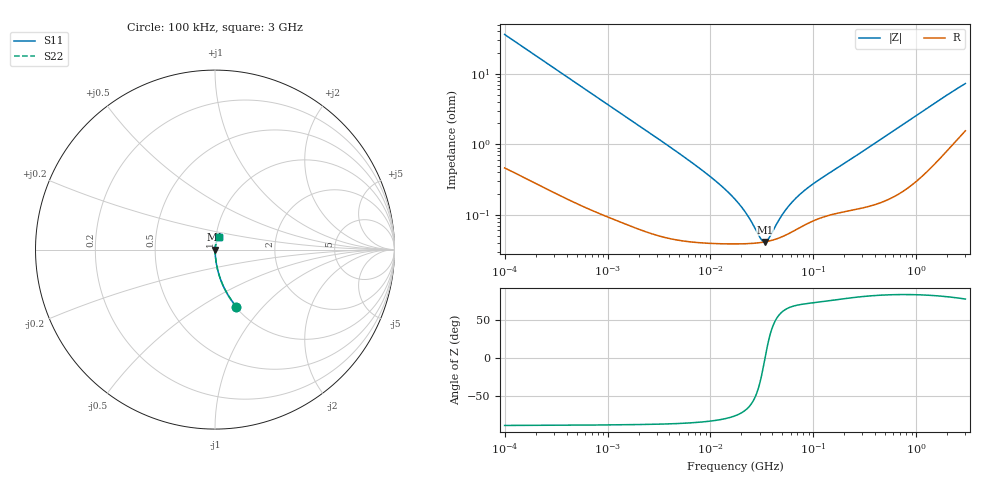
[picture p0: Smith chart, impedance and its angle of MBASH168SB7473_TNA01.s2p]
! MBASH168SB7473_TNA01  S-PARAMETER MODEL  ( Standard Model )
! Model Generated by TAIYO YUDEN Corporation (http://www.ty-top.com)
! Version 1.0
! TAIYO YUDEN Control No. 220601
! Copyright(c) 2016 TAIYO YUDEN CO.,LTD. All Rights Reserved.
! Product Description (link to TY-COMPAS)
! https://ds.yuden.co.jp/TYCOMPAS/or/detail?pn=MBASH168SB7473KTNA01&u=M
! Products Name : Multilayer Ceramic Capacitors
! Characteristics :
!  Capacitance : 0.047 [uF] , Rated Voltage : 100 [V] , TCC : X7R
!  Case Size : 1.6 x 0.8 / 0.063 x 0.031 [mm/inch] , Thickness : 0.8 / 0.031 [mm/inch]
!  (Conditions: Temperature = 25 [degC] , DC Bias Voltage = 0 [V])
! External Node Assignments :
!  1  o---| |---o  2
! GND o---------o GND
! Frequency Range : 100kHz  -  3GHz  [ 401 STEP ]
# MHZ S RI R 50
! Freq[MHz].  S11 Real  S11 Imag  S21 Real  S21 Imag  S12 Real  S12 Imag  S22 Real  S22 Imag
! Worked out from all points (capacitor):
!   401 points, 100 kHz to 3 GHz, reference 50 ohm
!   read as one part in series: C = 43.8 nF near 105.3 kHz
!   lowest |Z| = 41.2 mohm at 33.85 MHz (marker M1)
!   series resonance near 33.94 MHz, so ESL is about 500 pH
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0.1  0.1192 -0.3177  0.8808 0.3177  0.8808 0.3177  0.1192 -0.3177
0.147195  0.0604 -0.2312  0.9396 0.2312  0.9396 0.2312  0.0604 -0.2312
0.228123  0.0273 -0.1552  0.9727 0.1552  0.9727 0.1552  0.0273 -0.1552
0.562235  0.00558 -0.065  0.9944 0.065  0.9944 0.065  0.00558 -0.065
1.18716  0.00181 -0.0311  0.9982 0.0311  0.9982 0.0311  0.00181 -0.0311
3.161081  0.000639 -0.0118  0.9994 0.0118  0.9994 0.0118  0.000639 -0.0118
9.574722  0.000407 -0.00362  0.9996 0.00362  0.9996 0.00362  0.000407 -0.00362
13.7349  0.000392 -0.0023  0.9996 0.0023  0.9996 0.0023  0.000392 -0.0023
17.7727  0.000388 -0.00155  0.9996 0.00155  0.9996 0.00155  0.000388 -0.00155
22.99754  0.00039 -0.000892  0.9996 0.000892  0.9996 0.000892  0.00039 -0.000892
30.53531  0.000403 -0.000237  0.9996 0.000237  0.9996 0.000237  0.000403 -0.000237
32.15051  0.000407 -0.000121  0.9996 0.000121  0.9996 0.000121  0.000407 -0.000121
33.85116  0.000412 -5.56e-06  0.9996 5.56e-06  0.9996 5.56e-06  0.000412 -5.56e-06
35.64176  0.000418 0.00011  0.9996 -0.00011  0.9996 -0.00011  0.000418 0.00011
37.52708  0.000425 0.000226  0.9996 -0.000226  0.9996 -0.000226  0.000425 0.000226
47.32384  0.000474 0.000754  0.9995 -0.000754  0.9995 -0.000754  0.000474 0.000754
58.15973  0.000545 0.00124  0.9995 -0.00124  0.9995 -0.00124  0.000545 0.00124
73.34282  0.000656 0.00181  0.9993 -0.00181  0.9993 -0.00181  0.000656 0.00181
97.38194  0.000812 0.00256  0.9992 -0.00256  0.9992 -0.00256  0.000812 0.00256
547.5153  0.00187 0.0141  0.9981 -0.0141  0.9981 -0.0141  0.00187 0.0141
1746.113  0.0084 0.0431  0.9916 -0.0431  0.9916 -0.0431  0.0084 0.0431
3000  0.0202 0.0688  0.9798 -0.0688  0.9798 -0.0688  0.0202 0.0688
